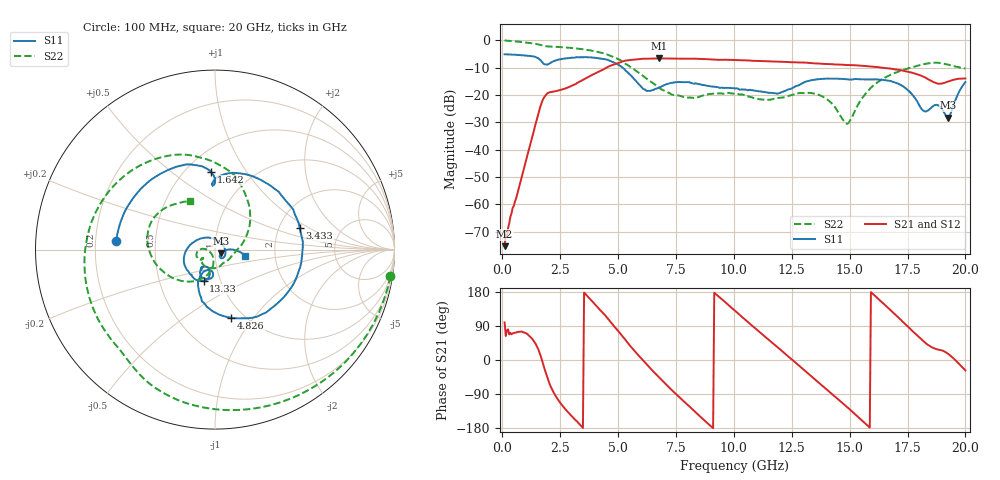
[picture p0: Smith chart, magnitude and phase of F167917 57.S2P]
!  2-Port S-parameters saved by WinCal
! VAR MeasName=S-Parameters (CALIBRATED_DATA) read from VNA (N5242A)
! VAR MeasDate=2016-11-22 9:02:48
! VAR NAME=F167917 57
! VAR FILENAME=F167917 57.S2P
! VAR DATE=2016-11-22 9:02:48
! VAR PHYS_PORTS=1,2
# Hz S DB R 50
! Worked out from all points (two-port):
!   401 points, 100 MHz to 20 GHz, reference 50 ohm
!   highest |S21| = -6.65 dB at 6.766 GHz (marker M1); lowest = -75.3 dB at 100 MHz (marker M2)
!   |S21| within 3 dB of the highest: 4.581 GHz to 15.95 GHz (11.37 GHz wide, 111 % of centre)
!   lowest |S11| = -28.3 dB at 19.25 GHz (marker M3), VSWR 1.08, Z = 53.3 - j2.24 ohm
!   |S11| at or under -10 dB: 5.19 GHz to end of sweep
!   |S22| runs from -30.6 to -0.1 dB; largest |S21 - S12| = 0.0044
!   S11 on the Smith chart (normalised r, x): 100 MHz: 0.29, +0.04; 1.642 GHz: 0.66, +0.70; 3.433 GHz: 2.60, +0.82; 4.826 GHz: 0.87, -0.78; 13.33 GHz: 0.83, -0.30; 20 GHz: 1.40, -0.10
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1e8  -5.16 175.1  -75.29 99.2  -75.05 69.0  -0.10 -8.7
8.4625e8  -5.48 138.5  -49.74 75.2  -49.68 73.8  -0.67 -66.9
1.64225e9  -7.24 92.9  -24.31 13.7  -24.31 13.7  -1.72 -119.1
2.5875e9  -6.82 65.9  -18.00 -119.6  -18.01 -119.6  -2.56 -163.3
3.43325e9  -6.25 14.2  -14.73 -175.9  -14.73 -175.7  -3.25 158.1
4.82625e9  -8.19 -76.8  -8.87 89.1  -8.83 89.1  -6.24 90.6
5.871e9  -15.86 -118.8  -6.96 12.9  -6.94 12.9  -11.73 40.8
6.7665e9  -17.36 -94.7  -6.65 -45.6  -6.65 -45.6  -17.35 4.6
7.662e9  -15.27 -108.3  -6.78 -98.9  -6.77 -98.8  -20.32 -31.7
8.60725e9  -16.30 -123.1  -6.86 -152.6  -6.83 -152.6  -20.36 -72.5
1.005e10  -17.64 -126.2  -7.26 129.9  -7.26 129.9  -19.59 -130.4
1.099525e10  -18.57 -125.3  -7.58 80.0  -7.55 79.9  -21.40 -146.6
1.199025e10  -19.26 -109.1  -7.87 28.4  -7.83 28.3  -21.09 -143.2
1.33335e10  -14.64 -110.1  -8.39 -42.6  -8.31 -42.4  -19.31 -163.4
1.338325e10  -14.60 -110.8  -8.38 -45.3  -8.33 -45.0  -19.37 -164.7
1.487575e10  -14.28 -132.3  -9.08 -123.4  -8.99 -123.8  -30.57 -143.1
1.5821e10  -14.33 -142.3  -9.53 -175.6  -9.52 -175.7  -18.25 -102.2
1.67165e10  -14.83 -163.7  -10.33 134.5  -10.39 134.3  -12.86 -128.3
1.8209e10  -25.87 62.5  -13.41 48.3  -13.38 48.6  -8.77 -178.1
1.875625e10  -23.62 -39.6  -15.78 28.5  -15.71 28.9  -8.23 158.6
1.925375e10  -28.29 -33.0  -15.12 16.3  -15.03 16.6  -8.94 138.1
2e10  -15.32 -11.3  -13.99 -27.4  -13.92 -27.1  -10.38 116.9
